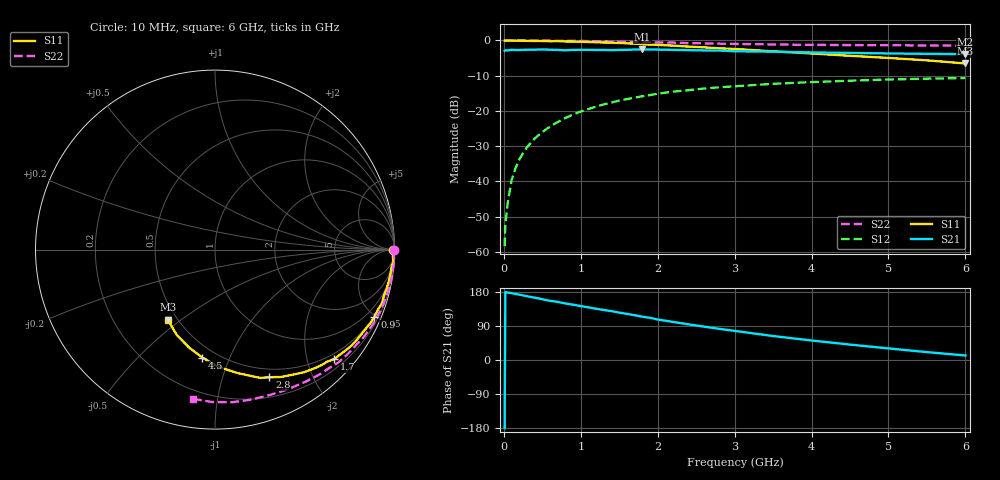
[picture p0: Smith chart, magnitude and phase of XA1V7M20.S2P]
! SIEMENS Discrete & RF Semiconductors
! BFY180
! Si NPN RF Bipolar Junction Transistor in MICRO-X
! VCE = 1.75 V  IC = 0.2 mA
! Common Emitter S-Parameters:  May  1997
# GHz  S  MA  R  50
!  f  S11  S21  S12  S22
! GHz  MAG  ANG  MAG  ANG  MAG  ANG  MAG  ANG
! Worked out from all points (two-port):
!   36 points, 10 MHz to 6 GHz, reference 50 ohm
!   highest |S21| = -2.53 dB at 1.8 GHz (marker M1); lowest = -3.9 dB at 6 GHz (marker M2)
!   |S21| within 3 dB of the highest: start of sweep to end of sweep
!   lowest |S11| = -6.5 dB at 6 GHz (marker M3), VSWR 2.78, Z = 22.3 - j22.3 ohm
!   |S11| at or under -10 dB: nowhere
!   |S22| runs from -1.5 to 0.0 dB; largest |S21 - S12| = 0.74
!   S11 on the Smith chart (normalised r, x): 10 MHz: open; 900 MHz: 0.47, -4.92; 1.7 GHz: 0.39, -2.51; 2.8 GHz: 0.41, -1.43; 4.5 GHz: 0.42, -0.80; 6 GHz: 0.45, -0.45
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0.01  0.9931 -0.1  0.714 -180.0  0.0012 94.0  0.9993 -0.2
0.02  0.9902 -0.4  0.727 179.3  0.0025 92.3  0.9999 -0.5
0.05  0.9909 -1.1  0.722 178.1  0.0049 88.5  0.9999 -1.0
0.1  0.9915 -2.4  0.738 176.4  0.0103 90.6  0.9966 -2.0
0.15  0.9964 -4.0  0.731 174.4  0.0152 88.0  0.9999 -3.0
0.2  0.9896 -5.0  0.732 172.5  0.0202 87.1  0.9997 -4.0
0.3  0.9871 -7.5  0.738 168.3  0.0304 83.4  0.9974 -6.1
0.4  0.9847 -10.1  0.739 164.6  0.0405 81.8  0.9987 -8.1
0.5  0.9813 -12.7  0.746 160.5  0.0501 79.2  0.9958 -10.1
0.7  0.9772 -17.8  0.733 153.3  0.0694 74.3  0.9911 -14.1
0.9  0.9639 -22.8  0.736 145.9  0.0889 70.1  0.9858 -18.2
1.1  0.9495 -27.4  0.736 138.8  0.1063 65.8  0.9783 -22.1
1.3  0.9359 -32.8  0.733 132.0  0.1239 61.3  0.9708 -26.1
1.7  0.9015 -42.6  0.744 118.2  0.1539 53.2  0.95 -33.7
1.8  0.8835 -45.0  0.747 114.2  0.1616 51.4  0.9464 -35.5
2.2  0.8445 -54.0  0.735 100.5  0.1877 43.5  0.9311 -42.7
2.8  0.7729 -66.9  0.72 82.3  0.2162 33.5  0.9007 -52.3
3.5  0.7001 -79.5  0.693 63.2  0.2424 23.4  0.8779 -62.5
4  0.6537 -88.4  0.676 51.5  0.2564 16.6  0.8653 -69.6
4.5  0.6054 -96.7  0.665 40.7  0.2681 10.5  0.8595 -76.7
5.5  0.5219 -114.0  0.645 20.8  0.2868 -1.4  0.8493 -91.1
6  0.471 -124.0  0.639 11.9  0.2927 -7.4  0.8406 -98.3
